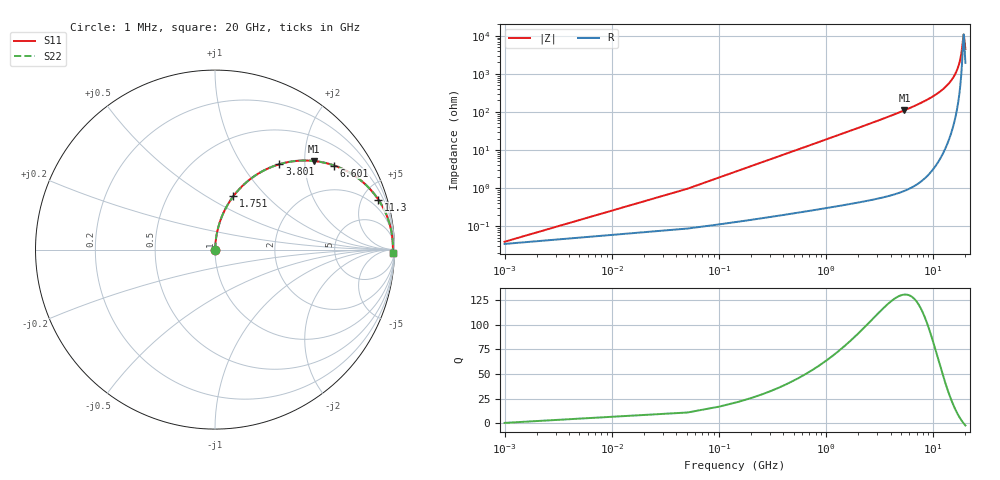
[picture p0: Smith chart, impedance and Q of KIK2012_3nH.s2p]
!version-2
!date-01.2022
!Series
# MHz S RI R 50
!Freq ReS11 ImS11 ReS21 ImS21 ReS12 ImS12 ReS22 ImS22
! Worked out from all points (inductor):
!   401 points, 1 MHz to 20 GHz, reference 50 ohm
!   read as one part in series: L = 3 nH near 101 MHz
!   highest Q = 131 at 5.401 GHz (marker M1), where L = 3.26 nH
!   self-resonance near 19.25 GHz
!   S11 on the Smith chart (normalised r, x): 1 MHz: 1.00, +0.00; 1.751 GHz: 1.01, +0.67; 3.801 GHz: 1.01, +1.49; 6.601 GHz: 1.02, +2.82; 11.3 GHz: 1.10, +6.49; 20 GHz: 40, -80
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1  0.000342 0.000188  0.9997 -0.000188  0.9997 -0.000188  0.000342 0.000188
151  0.00211 0.0284  0.9979 -0.0284  0.9979 -0.0284  0.00211 0.0284
251  0.00383 0.0471  0.9962 -0.0471  0.9962 -0.0471  0.00383 0.0471
351  0.00619 0.0657  0.9938 -0.0657  0.9938 -0.0657  0.00619 0.0657
551  0.0129 0.1024  0.9871 -0.1024  0.9871 -0.1024  0.0129 0.1024
851  0.0277 0.1558  0.9723 -0.1558  0.9723 -0.1558  0.0277 0.1558
1751  0.1025 0.2975  0.8975 -0.2975  0.8975 -0.2975  0.1025 0.2975
3351  0.2995 0.4537  0.7005 -0.4537  0.7005 -0.4537  0.2995 0.4537
3801  0.3583 0.4754  0.6417 -0.4754  0.6417 -0.4754  0.3583 0.4754
5401  0.5493 0.4937  0.4507 -0.4937  0.4507 -0.4937  0.5493 0.4937
6601  0.664 0.4684  0.336 -0.4684  0.336 -0.4684  0.664 0.4684
6701  0.6724 0.4654  0.3276 -0.4654  0.3276 -0.4654  0.6724 0.4654
10001  0.8664 0.3342  0.1336 -0.3342  0.1336 -0.3342  0.8664 0.3342
11301  0.9097 0.2788  0.0903 -0.2788  0.0903 -0.2788  0.9097 0.2788
13351  0.9541 0.1961  0.0459 -0.1961  0.0459 -0.1961  0.9541 0.1961
15251  0.9772 0.1263  0.0228 -0.1263  0.0228 -0.1263  0.9772 0.1263
16701  0.9866 0.0776  0.0134 -0.0776  0.0134 -0.0776  0.9866 0.0776
18151  0.9906 0.0326  0.00938 -0.0326  0.00938 -0.0326  0.9906 0.0326
18551  0.991 0.0208  0.00904 -0.0208  0.00904 -0.0208  0.991 0.0208
19201  0.9909 0.00217  0.0091 -0.00217  0.0091 -0.00217  0.9909 0.00217
19401  0.9907 -0.00342  0.00926 0.00342  0.00926 0.00342  0.9907 -0.00342
20000  0.9899 -0.0198  0.0101 0.0198  0.0101 0.0198  0.9899 -0.0198
